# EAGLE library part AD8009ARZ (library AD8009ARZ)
AD8009ARZ, Fast Operational Amplifier Current Feedback,, 9V, 8-Pin SOIC Source: Datasheet
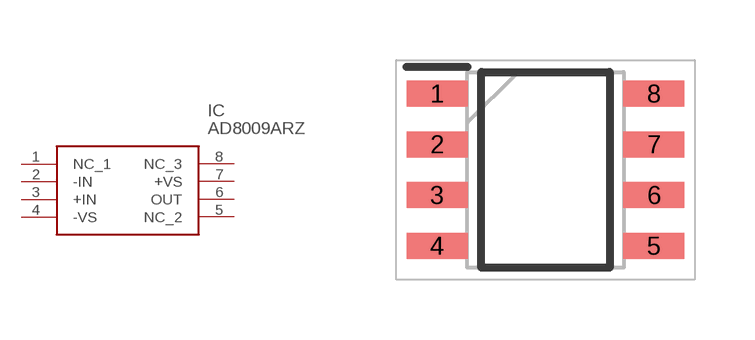
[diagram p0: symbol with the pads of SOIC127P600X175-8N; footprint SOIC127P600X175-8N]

Designator prefix IC

## AD8009ARZ (Description: AD8009ARZ, Fast Operational Amplifier Current Feedback,, 9V, 8-Pin SOIC; Height: 1.75mm; Manufacturer_Name: Analog Devices; Manufacturer_Part_Number: AD8009ARZ; Mouser_Part_Number: 584-AD8009ARZ; Mouser_Price-Stock: https://www.mouser.co.uk/ProductDetail/Analog-Devices/AD8009ARZ?qs=%2FtpEQrCGXCztmOs2ZWYkdw%3D%3D)  [SOIC127P600X175-8N]
1  NC_1
2  -IN
3  +IN
4  -VS
5  NC_2
6  OUT
7  +VS
8  NC_3

## Footprint SOIC127P600X175-8N (pad centres in mm)
R-8 (SOIC)
smd 1.525 x 0.65: 1 -2.712,1.905; 2 -2.712,0.635; 3 -2.712,-0.635; 4 -2.712,-1.905; 5 2.712,-1.905; 6 2.712,-0.635; 7 2.712,0.635; 8 2.712,1.905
